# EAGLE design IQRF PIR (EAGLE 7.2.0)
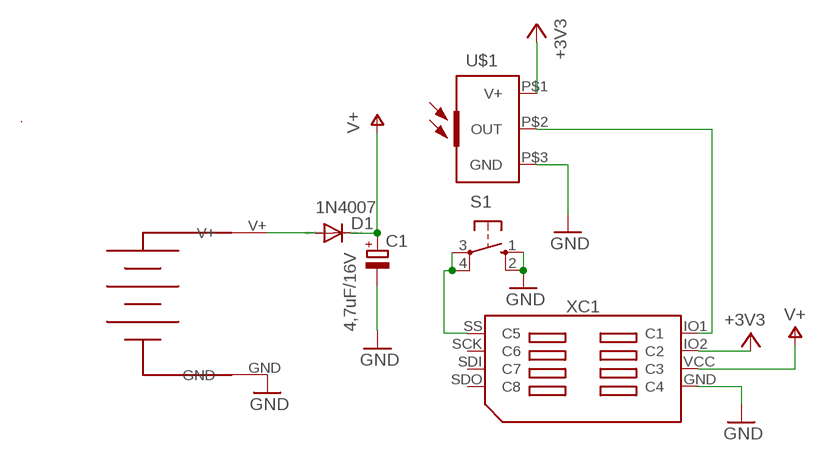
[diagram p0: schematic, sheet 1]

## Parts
3XAA1,5V  3AA  [3AA]
C1  4,7uF/16V  CPOL-EUE2,5-6E  [E2,5-6E]
D1  1N4007  DIODE-DO34-7  [DO34-7]
S1  10-XX  [B3F-10XX]
U$1  E332  [LINE]
XC1  SIM8X_KON-SIM02  [SIM_02]

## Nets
+3V3: U$1.P$1(V+) XC1.IO2(C2)
GND: 3XAA1,5V.GND C1.- S1.1(S) S1.2(S1) U$1.P$3(GND) XC1.GND(C4)
N$1: 3XAA1,5V.V+ D1.A
N$4: U$1.P$2(OUT) XC1.IO1(C1)
N$5: S1.3(P) S1.4(P1) XC1.SS(C5)
V+: C1.+ D1.C XC1.VCC(C3)
Unconnected: XC1.SCK(C6) XC1.SDI(C7) XC1.SDO(C8)

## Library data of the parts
3XAA1,5V = battery:3AA
C1 = rcl:CPOL-EU: POLARIZED CAPACITOR, European symbol
D1 = diode:DIODE-: DIODE
S1 = switch-omron:10-XX: OMRON SWITCH; MPN: B3F-1000; OC_FARNELL: 176432; OC_NEWARK: 36M3542
U$1 = sensor-infratec:E332
XC1 = KON-SIM-02_150624:SIM8X_KON-SIM: KON-SIM-02

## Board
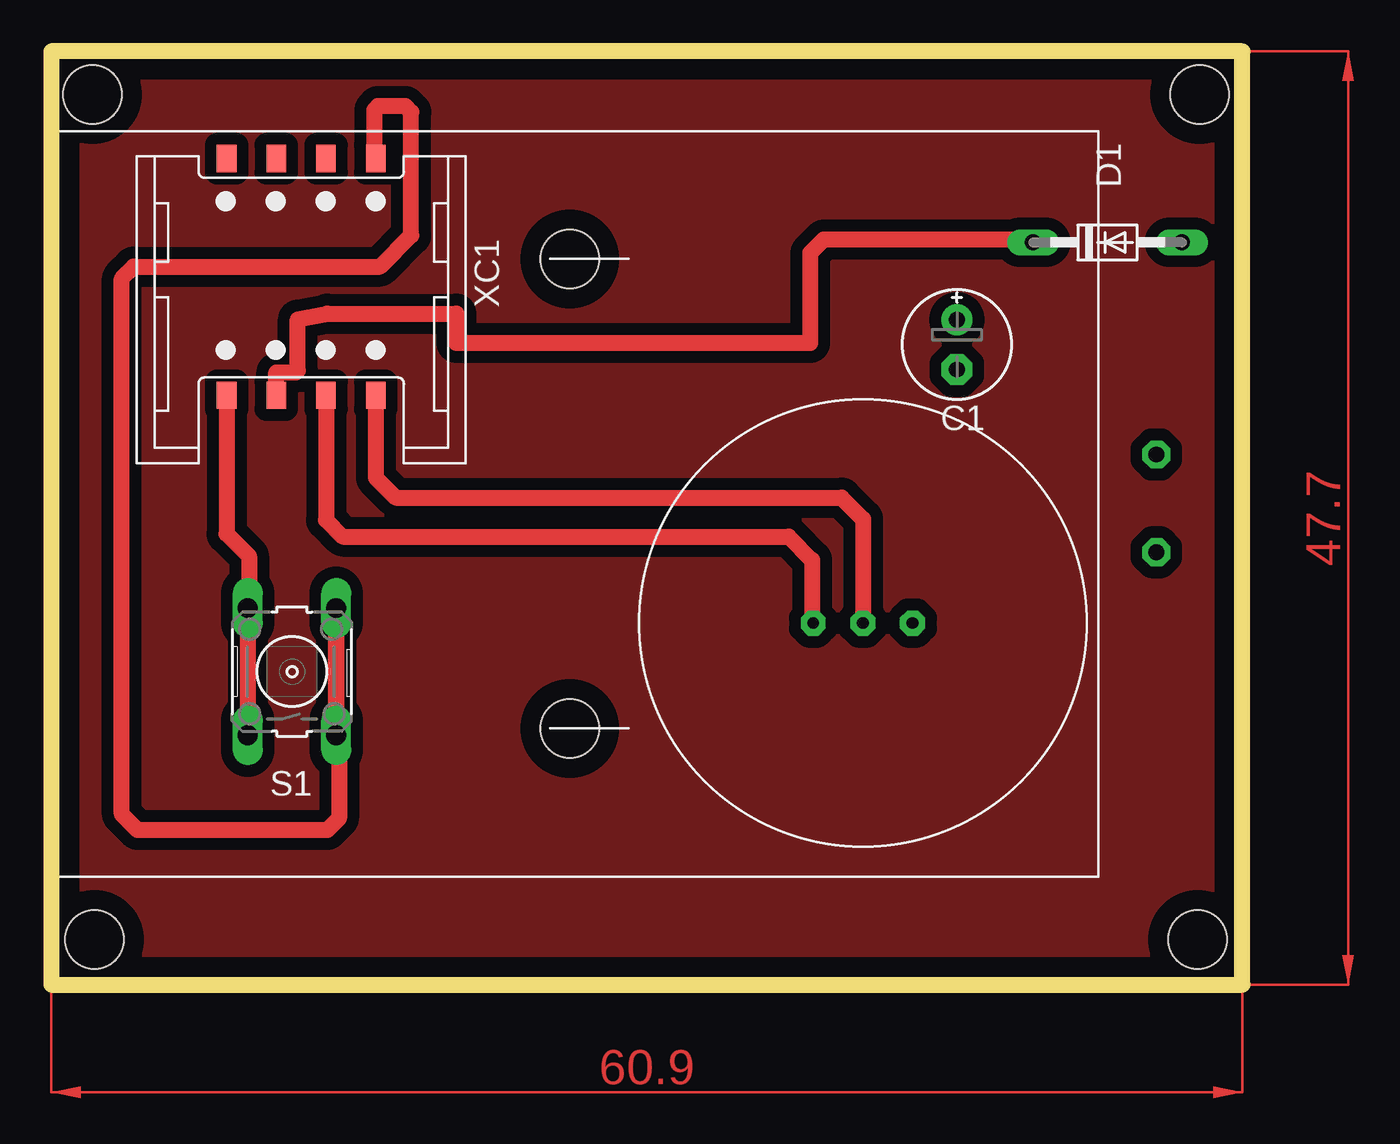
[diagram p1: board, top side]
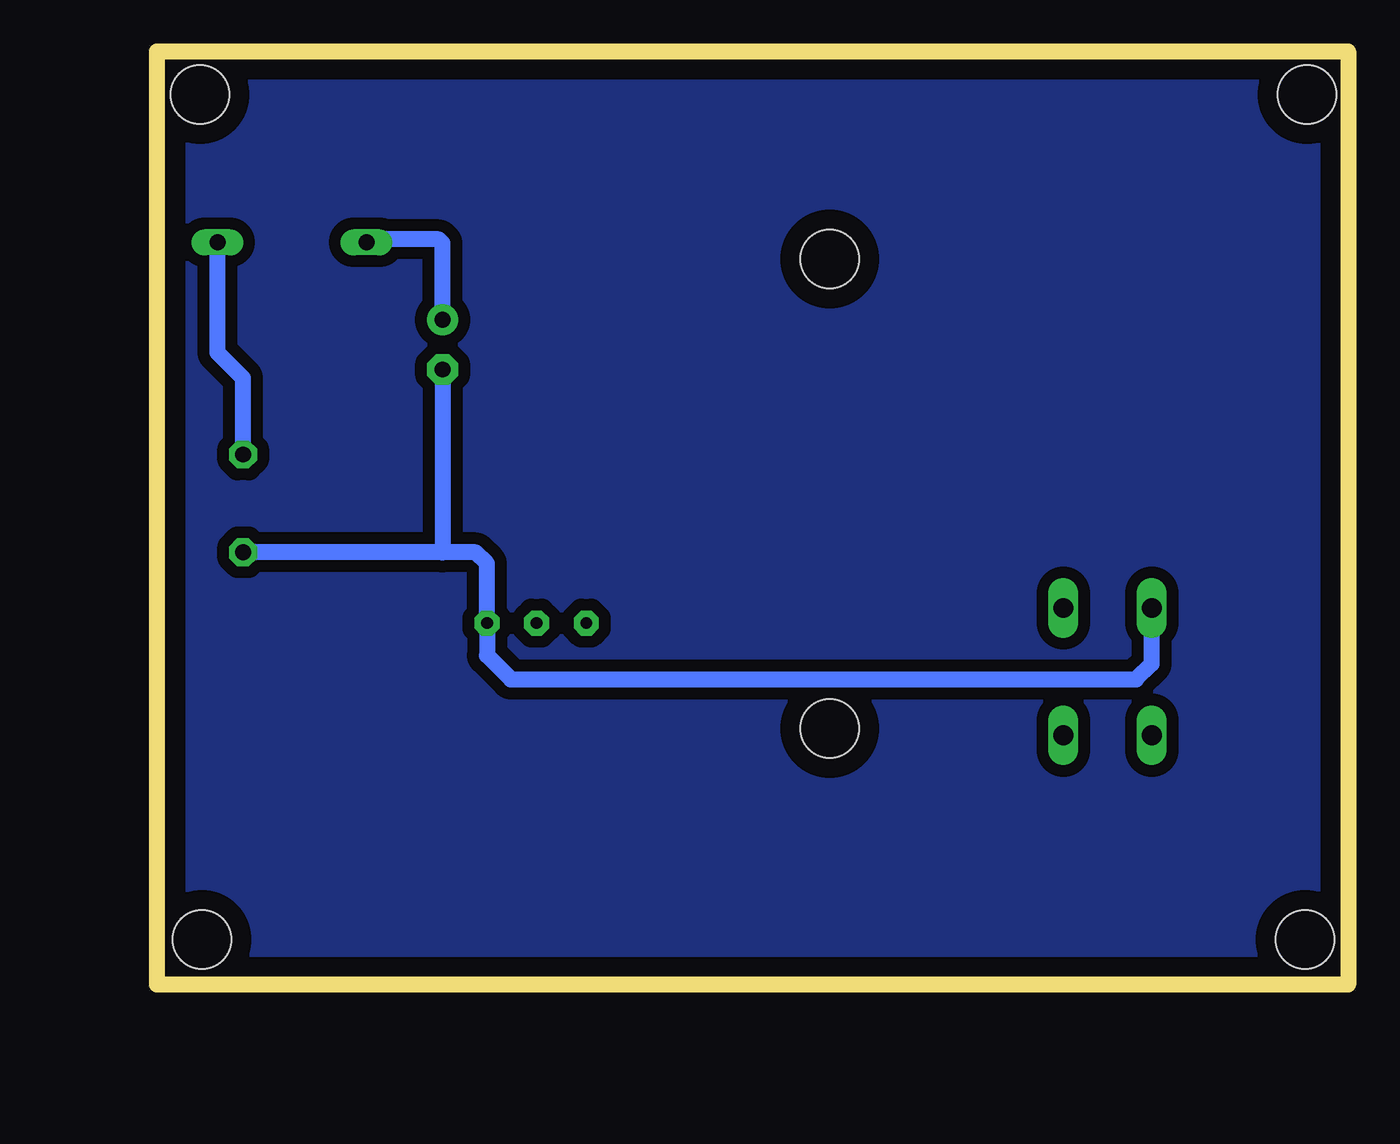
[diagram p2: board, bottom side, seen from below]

Size 60.9 x 47.7 mm. Coordinates in mm from the lower left corner, seen from the top.
Outline: 0,0 60.9,0 60.9,47.7 0,47.7 0,0
Copper layers (1*16): Top 0.035mm / dielectric 1.5mm / Bottom 0.035mm
Design rules "default": minimum track width 10mil, minimum drill 24mil, track to track 8mil, track to pad 8mil, pad to pad 8mil, via to via 8mil, smd to smd 8mil, copper to edge 40mil, drill to drill 8mil, minimum pad ring 10mil, minimum via ring 8mil, stop-mask expansion 4mil, vias tented up to drill 0mil, thermal gap 10mil
Holes 3 mm at 2.2,2.3 2.1,45.5 58.7,45.5 58.6,2.3

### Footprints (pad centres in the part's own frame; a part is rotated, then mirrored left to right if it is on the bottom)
3AA = drill 0.8 pad 1.422 octagon: GND 36,-5; V+ 36,0 | hole 3: 6,10; 6,-14
E2,5-6E = drill 0.813 pad 1.575: + -1.27,0 | drill 0.813 pad 1.575 octagon: - 1.27,0
DO34-7 = drill 0.813 long: A 3.81,0; C -3.81,0
B3F-10XX = drill 1.016 long: 1 -3.251,2.261; 2 3.251,2.261; 3 -3.251,-2.261; 4 3.251,-2.261
LINE = drill 0.6 pad 1.27 octagon: P$1 -6.35,5.08; P$2 -3.81,5.08; P$3 -1.27,5.08
SIM_02 = smd 1.4 x 1: GND 6.112,-3.81; IO1 6.112,3.81; IO2 6.112,1.27; SCK -5.98,1.27; SDI -5.98,-1.27; SDO -5.98,-3.81; SS -5.98,3.81; VCC 6.112,-1.27

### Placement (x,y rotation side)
3XAA1,5V  20.5,27.1 0 top
C1  46.3,32.71 270 top
D1  54,37.94 0 top
S1  12.3,16 90 top
U$1  45.3,13.4 0 top
XC1  12.77,36.24 270 top

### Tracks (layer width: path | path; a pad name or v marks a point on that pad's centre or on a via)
+3V3
  Top 0.813: XC1.IO2 14.04,23.76 14.9,22.9 37.7,22.9 38.9,21.7 38.9,18.53 U$1.P$1
GND
  Top 0.813: XC1.GND 8.96,23.04 10.1,21.9 10.1,19.31 S1.2 S1.1
  Bottom 0.813: S1.2 10.04,16.4 10.84,15.6 42.8,15.6 44.03,16.83 U$1.P$3 44.03,21.53 44.6,22.1 46.3,22.1 | 46.3,22.1 3XAA1,5V.GND | C1.- 46.3,22.1
N$1
  Bottom 0.813: 3XAA1,5V.V+ 56.5,31 57.8,32.3 D1.A
N$2
  pour Top (isolate 0.61): 0.7,3.7 0.7,43.5 3.8,46.5 57,46.5 59.9,43.6 59.9,3.6 56.9,0.6 3.8,0.6
N$4
  Top 0.813: XC1.IO1 16.58,25.92 17.6,24.9 40.4,24.9 41.5,23.8 U$1.P$2
N$5
  Top 0.813: S1.3 S1.4 14.56,12.94 14.7,12.8 14.7,8.5 14.1,7.9 4.4,7.9 3.6,8.7 3.6,36.1 4.2,36.7 16.8,36.7 18.4,38.3 18.4,44.6 18.1,44.9 16.7,44.9 16.5,44.7 16.5,42.3 XC1.SS
N$6
  pour Bottom (isolate 0.61): 3.8,0.6 56.9,0.6 59.9,3.6 59.9,43.6 57,46.5 3.7,46.5 0.7,43.5 0.7,3.7
V+
  Top 0.813: XC1.VCC 11.5,31.3 12.5,31.3 12.6,31.4 12.6,34 14.1,34.3 20.7,34.3 20.7,32.8 38.8,32.8 38.8,35.5 38.8,37.4 39.5,38.1 50.03,38.1 D1.C
  Bottom 0.813: C1.+ 46.3,37.9 46.5,38.1 50.03,38.1 D1.C
(copper drawn outside any net)
  shapes: Top area x2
